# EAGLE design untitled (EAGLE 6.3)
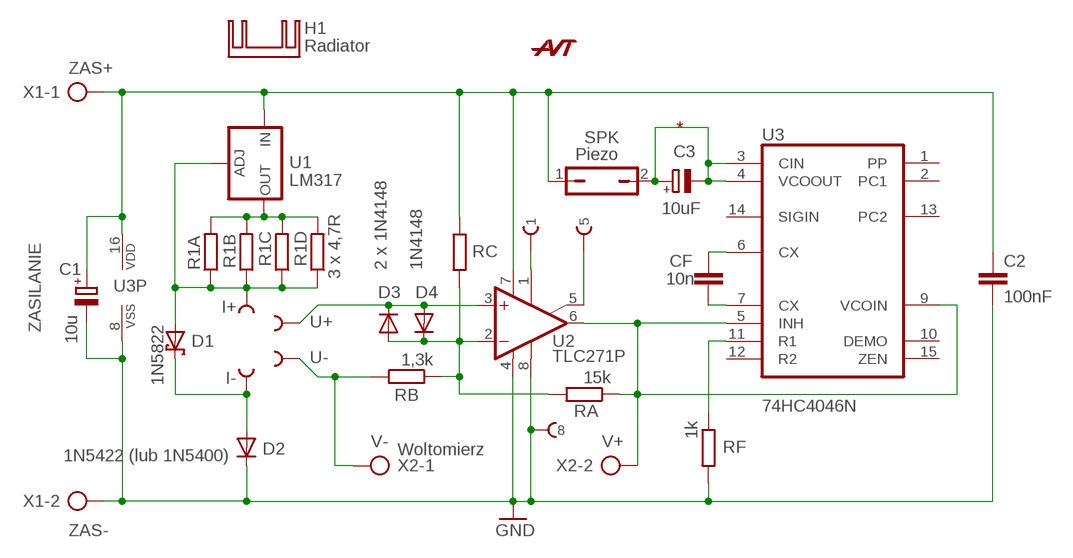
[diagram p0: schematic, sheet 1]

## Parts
1  2.5/1  [2.5/1]
5  2.5/1  [2.5/1]
8  2.5/1  [2.5/1]
C1  10u  CPOL-EUE3.5-8  [E3,5-8]
C2  100nF  C-EU050-030X075  [C050-030X075]
C3  10uF  CPOL-EUE3,5-6  [E3,5-6]
CF  10n  C-EU050-055X075  [C050-055X075]
D1  1N5822  1N5822-17.5  [DO201T17.5]
D2  1N5422 (lub 1N5400)  1N5400-17.5  [DO201-17.5]
D3  2 x 1N4148  1N4148DO35-10  [DO35-10]
D4  1N4148  1N4148DO35-10  [DO35-10]
H1  Radiator  RAD_DY-CN_20MM  [RAD_DY-CN_20MM]
I+  3.5/1.5  [3.5/1.5]
I-  3.5/1.5  [3.5/1.5]
R1A  R-EU_0207/10  [0207/10]
R1B  R-EU_0207/10  [0207/10]
R1C  R-EU_0207/10  [0207/10]
R1D  3 x 4,7R  R-EU_0207/10  [0207/10]
RA  15k  R-EU_0207/10  [0207/10]
RB  1,3k  R-EU_0207/10  [0207/10]
RC  R-EU_0207/10  [0207/10]
RF  1k  R-EU_0207/10  [0207/10]
SPK  Piezo  JP1Q  [JP1]
U1  LM317  LM317TS  [317TS]
U2  TLC271P  [DIL08]
U3  74HC4046N  4046N  [DIL16]
U$1  LOGOSMALL  [SIZE_S]
U+  3.5/1.5  [3.5/1.5]
U-  3.5/1.5  [3.5/1.5]
X1  ZASILANIE  AK500/2  [AK500/2]
X2  Woltomierz  AK500/2  [AK500/2]

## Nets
GND: 8.1(P) C1.- C2.2 D2.C RF.2 U2.4(V-) U2.8(OPT) U3.8(VSS) X1.2
N$1: R1A.2 R1B.2 R1C.2 R1D.2 U1.2(OUT)
N$2: D1.A I+.1(P) R1A.1 R1B.1 R1C.1 R1D.1 U1.1(ADJ)
N$3: D1.C D2.A I-.1(P)
N$5: C1.+ C2.1 RC.1 SPK.1 U1.3(IN) U2.7(V+) U3.16(VDD) X1.1
N$6: D3.C D4.A U2.3(+IN) U+.1(P)
N$7: RA.1 U2.6(OUT) U3.5(INH) U3.9(VCOIN) X2.2
N$8: D3.A D4.C RA.2 RB.1 RC.2 U2.2(-IN)
N$9: RB.2 U-.1(P) X2.1
N$10: C3.+ C3.- SPK.2 U3.3(CIN) U3.4(VCOOUT)
N$11: RF.1 U3.11(R1)
N$12: CF.1 U3.6(CX)
N$13: CF.2 U3.7(CX)
N$14: 1.1(P) U2.1(ON1)
N$15: 5.1(P) U2.5(ON2)
Unconnected: U3.1(PP) U3.2(PC1) U3.10(DEMO) U3.12(R2) U3.13(PC2) U3.14(SIGIN) U3.15(ZEN)

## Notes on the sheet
- ZAS+
- *
- V- | V+
- ZAS-

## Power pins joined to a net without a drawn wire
P$1: H1.P$1

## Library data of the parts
1 5 8 = wirepad:2.5/1
C1 C3 = rcl:CPOL-EU: POLARIZED CAPACITOR, European symbol
C2 CF = rcl:C-EU: CAPACITOR, European symbol
D1 = diode:1N5822: Diameter 5.6 mm, vertical, grid 10.16 mm
D2 = diode:1N5400: DIODE
D3 D4 = diode:1N4148: DIODE
H1 = radiator:RAD_DY-CN_20MM: Radiator, profil DY-CN; dl=20mm szer=15mm wys=11mm
I+ I- U+ U- = wirepad:3.5/1.5
R1A R1B R1C R1D RA RB RC RF = rcl:R-EU_: RESISTOR, European symbol
SPK = jumper:JP1Q: JUMPER
U1 = v-reg:LM317TS: VOLTAGE REGULATOR
U2 = linear:TLC271: OP AMP
U3 = 40xx:4046: Micropower PLL
U$1 = AVT_Logo:LOGO: Nowe Logo AVT
X1 X2 = con-ptr500:AK500/2: CONNECTOR; OC_FARNELL: unknown; OC_NEWARK: unknown

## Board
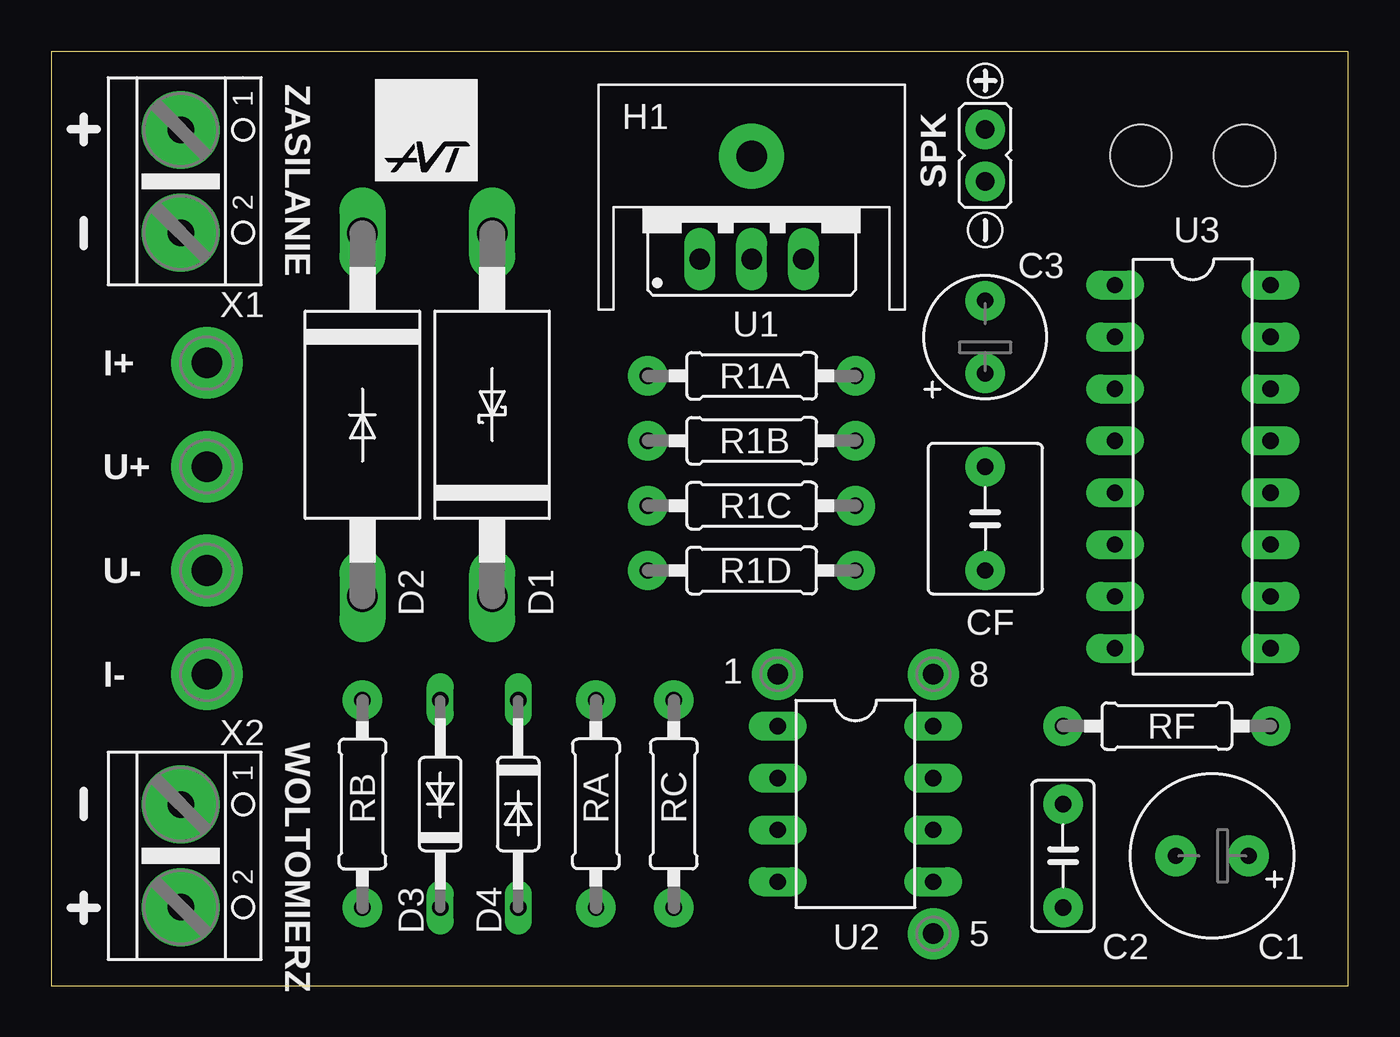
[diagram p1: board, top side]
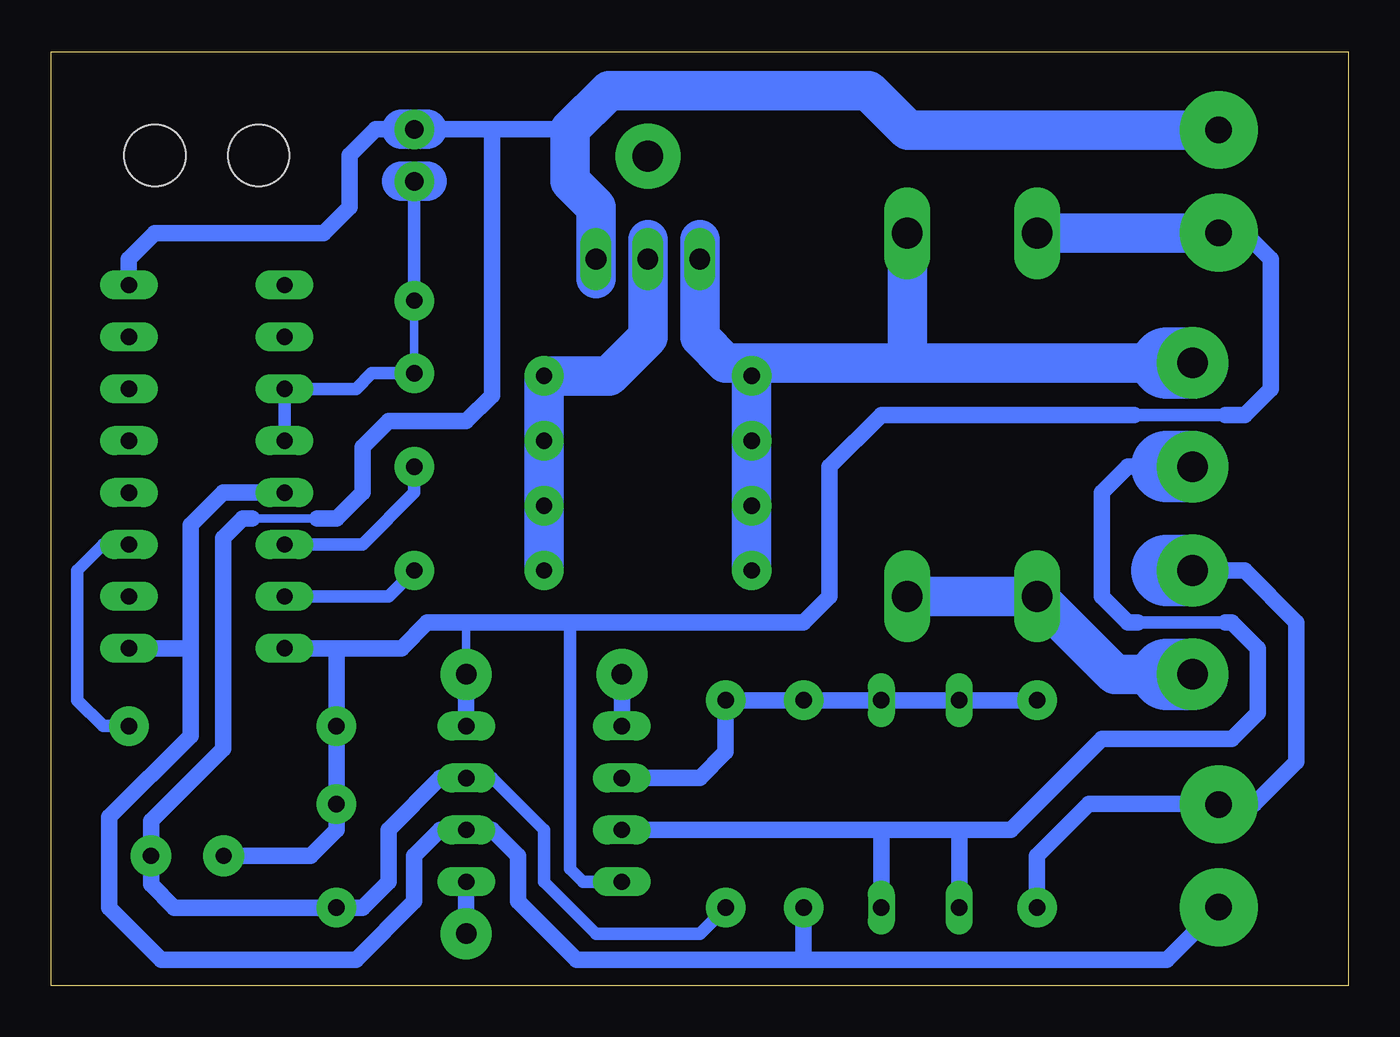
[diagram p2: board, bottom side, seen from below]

Size 63.5 x 45.72 mm. Coordinates in mm from the lower left corner, seen from the top.
Outline: 0,0 63.5,0 63.5,45.72 0,45.72 0,0
Copper layers (1*16): Top 0.035mm / dielectric 1.5mm / Bottom 0.035mm
Design rules "default": minimum track width 10mil, minimum drill 24mil, track to track 8mil, track to pad 8mil, pad to pad 8mil, via to via 8mil, smd to smd 8mil, copper to edge 40mil, drill to drill 8mil, minimum pad ring 10mil, minimum via ring 8mil, stop-mask expansion 4mil, vias tented up to drill 0mil, thermal gap 10mil
Holes 3 mm at 53.34,40.64 58.42,40.64

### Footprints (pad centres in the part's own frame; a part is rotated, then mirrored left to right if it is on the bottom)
2.5/1 = drill 1 pad 2.5: 1 0,0
E3,5-8 = drill 0.8 pad 2: + -1.778,0; - 1.778,0
C050-030X075 = drill 0.8 pad 1.93: 1 -2.54,0; 2 2.54,0
E3,5-6 = drill 0.8 pad 1.93: + -1.778,0; - 1.778,0
C050-055X075 = drill 0.8 pad 1.93: 1 -2.54,0; 2 2.54,0
DO201T17.5 = drill 1.499 long: A 8.89,0; C -8.89,0
DO201-17.5 = drill 1.499 long: A 8.89,0; C -8.89,0
DO35-10 = drill 0.813 long: A 5.08,0; C -5.08,0
RAD_DY-CN_20MM = drill 1.5 pad 3.175: P$1 0,-2.5
3.5/1.5 = drill 1.5 pad 3.5: 1 0,0
0207/10 = drill 0.8 pad 1.93: 1 -5.08,0; 2 5.08,0
JP1 = drill 0.914 pad 1.93: 1 0,-1.27; 2 0,1.27
317TS = drill 1.016 long: 1 -2.54,-2.54; 2 0,-2.54; 3 2.54,-2.54
DIL08 = drill 0.8 pad 1.422 long: 1 -3.81,-3.81; 2 -1.27,-3.81; 3 1.27,-3.81; 4 3.81,-3.81; 5 3.81,3.81; 6 1.27,3.81; 7 -1.27,3.81; 8 -3.81,3.81
DIL16 = drill 0.8 pad 1.422 long: 1 -8.89,-3.81; 2 -6.35,-3.81; 3 -3.81,-3.81; 4 -1.27,-3.81; 5 1.27,-3.81; 6 3.81,-3.81; 7 6.35,-3.81; 8 8.89,-3.81; 9 8.89,3.81; 10 6.35,3.81; 11 3.81,3.81; 12 1.27,3.81; 13 -1.27,3.81; 14 -3.81,3.81; 15 -6.35,3.81; 16 -8.89,3.81
AK500/2 = drill 1.3 pad 3.81: 1 -2.515,0; 2 2.515,0

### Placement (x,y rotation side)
1  35.56,15.24 0 top
5  43.18,2.54 0 top
8  43.18,15.24 0 top
C1  56.83,6.35 180 top
C2  49.53,6.35 90 top
C3  45.72,31.75 90 top
CF  45.72,22.86 270 top
D1  21.59,27.94 90 top
D2  15.24,27.94 270 top
D3  19.05,8.89 90 top
D4  22.86,8.89 270 top
H1  34.29,38.1 180 top
I+  7.62,30.48 0 top
I-  7.62,15.24 0 top
R1A  34.29,29.84 0 top
R1B  34.29,26.67 0 top
R1C  34.29,23.5 0 top
R1D  34.29,20.32 0 top
RA  26.67,8.89 90 top
RB  15.24,8.89 270 top
RC  30.48,8.89 90 top
RF  54.61,12.7 180 top
SPK  45.72,40.64 180 top
U1  34.29,38.1 0 top
U2  39.37,8.89 270 top
U3  55.88,25.4 270 top
U$1  15.88,39.37 0 top
U+  7.62,25.4 0 top
U-  7.62,20.32 0 top
X1  6.35,39.37 270 top
X2  6.35,6.35 270 top

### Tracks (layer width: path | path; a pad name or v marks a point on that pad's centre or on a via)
GND
  Bottom 0.406: 43.18,17.78 8.1 | 6.33,36.83 X1.2
  Bottom 0.61: U2.4 37.47,5.08 38.1,5.71 38.1,17.78 | 6.03,27.94 10.48,27.94
  Bottom 0.813: 8.1 U2.8 | 49.53,16.51 46.35,16.51 45.09,17.78 43.18,17.78 38.1,17.78 26.67,17.78 25.4,19.05 25.4,25.4 22.86,27.94 10.48,27.94 | 49.53,16.51 U3.8 | 49.53,16.51 RF.2 C2.2 49.53,7.62 50.8,6.35 C1.- | 6.33,36.83 5.08,36.83 3.81,35.56 3.81,29.21 5.08,27.94 6.03,27.94
  Bottom 1.27: X1.2 6.38,36.83
  Bottom 1.93: 6.38,36.83 D2.C
N$1
  Bottom 1.93: R1D.2 R1C.2 R1B.2 R1A.2 36.2,29.84 34.29,31.75 U1.2 34.29,36.51
N$2
  Bottom 1.93: R1D.1 R1C.1 R1B.1 R1A.1 29.21,30.48 | 29.21,30.48 30.48,30.48 31.75,31.75 U1.1 31.75,36.51 | 8.89,30.48 21.59,30.48 | 21.59,30.48 29.21,30.48 | 21.59,30.48 D1.A
  Bottom 3.5: I+.1 8.89,30.48
N$3
  Bottom 1.93: D1.C D2.A 11.43,15.24 8.89,15.24
  Bottom 3.5: I-.1 8.89,15.24
N$5
  Bottom 0.406: 53.66,22.86 50.48,22.86
  Bottom 0.61: RC.1 31.75,2.54 36.83,2.54 39.37,5.08 39.37,7.62 41.91,10.16 U2.7
  Bottom 0.813: 41.91,41.91 38.1,41.91 | 41.91,41.91 45.09,41.91 | 46.35,41.91 47.62,41.91 48.9,40.64 48.9,38.1 50.16,36.83 58.42,36.83 59.69,35.56 U3.16 | U2.7 44.45,10.16 46.99,7.62 46.99,5.08 48.26,3.81 C2.1 57.47,3.81 58.61,4.95 C1.+ 58.61,8.06 55.09,11.59 55.09,21.91 54.13,22.86 53.66,22.86 | 41.91,41.91 41.91,28.89 43.18,27.62 46.99,27.62 48.26,26.35 48.26,24.13 49.53,22.86 50.48,22.86
  Bottom 1.93: X1.1 21.57,41.88 23.5,43.81 36.2,43.81 38.1,41.91 38.1,39.37 36.83,38.1 U1.3 36.83,34.61 | 45.09,41.91 SPK.1 46.35,41.91
N$6
  Bottom 0.61: 6.03,17.78 10.32,17.78
  Bottom 0.813: 19.05,7.62 22.86,7.62 | 22.86,7.62 U2.3 | 19.05,7.62 D3.C | 22.86,7.62 D4.A | 19.05,7.62 16.51,7.62 12.06,12.06 5.71,12.06 4.45,13.34 4.45,16.51 5.71,17.78 6.03,17.78 | 10.32,17.78 10.79,17.78 12.06,19.05 12.06,24.13 10.79,25.4 U+.1
  Bottom 3.5: U+.1 8.89,25.4
N$7
  Bottom 0.406: X2.2 6.35,3.81
  Bottom 0.813: 6.35,3.81 8.89,1.27 26.67,1.27 | 26.67,1.27 37.78,1.27 40.64,4.13 40.64,6.35 41.91,7.62 U2.6 44.45,7.62 45.72,6.35 45.72,4.13 48.58,1.27 58.1,1.27 60.64,3.81 60.64,8.26 56.67,12.22 56.67,16.51 | 26.67,1.27 RA.1 | U3.5 55.09,24.13 56.67,22.54 56.67,16.51 | 56.67,16.51 U3.9
N$8
  Bottom 0.813: U2.2 31.75,10.16 30.48,11.43 RC.2 RA.2 D4.C D3.A RB.1
N$9
  Bottom 0.406: 6.33,8.89 X2.1 6.35,8.89
  Bottom 0.813: U-.1 5.08,20.32 2.54,17.78 2.54,10.95 4.6,8.89 6.33,8.89 | RB.2 15.24,6.35 12.7,8.89 6.35,8.89
  Bottom 3.5: U-.1 8.89,20.32
N$10
  Bottom 0.406: C3.+ C3.-
  Bottom 0.61: U3.4 U3.3 48.58,29.21 47.82,29.97 C3.+ | C3.- SPK.2
  Bottom 1.93: 45.09,39.37 SPK.2 46.35,39.37
N$11
  Bottom 0.61: U3.11 60.96,21.59 62.23,20.32 62.23,13.97 60.96,12.7 RF.1
N$12
  Bottom 0.61: U3.6 48.26,21.59 45.72,24.13 CF.1
N$13
  Bottom 0.61: U3.7 46.99,19.05 CF.2
N$14
  Bottom 0.813: U2.1 1.1
N$15
  Bottom 0.813: 5.1 U2.5

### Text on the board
tPlace: ZASILANIE | WOLTOMIERZ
